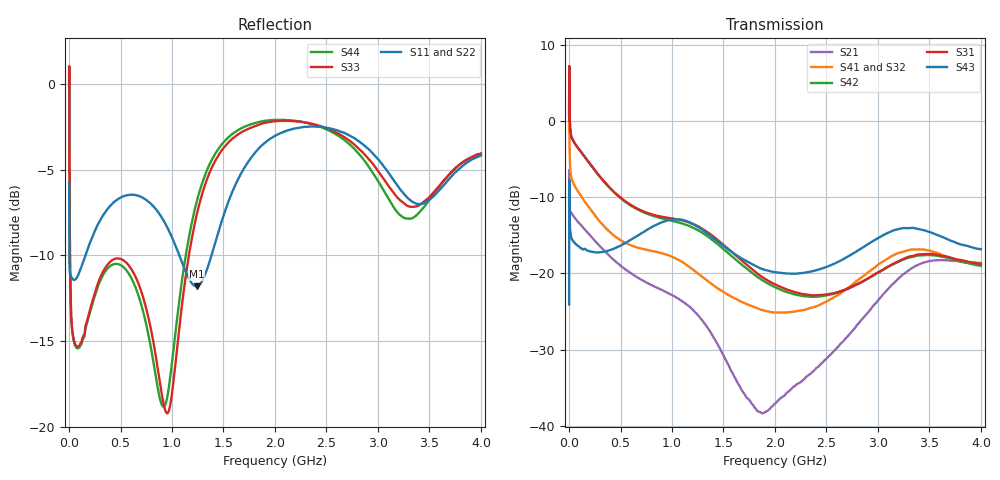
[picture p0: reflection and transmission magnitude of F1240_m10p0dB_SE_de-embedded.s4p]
! Integrated Device Technology
! Corporate Headquarters
! 6024 Silver Creek Valley Road
! San Jose, CA 95138  USA
! Phone:  1-408-284-8200
! Toll Free:  1-800-223-1366
! Webpage:  http://www.idt.com/
! Timing and RF Division
! 515 Groton Road, Suite 102
! Westford, MA 01886-6024
! Device:  F1240
! Description: Dual Intermediate Frequency Digital Variable Gain Amplifier
! Frequency:  10.0 -  500.00 MHz
! Package:  5x5 mm QFN Plastic Package: 32 pin
! Ports:  8 RF, 20 DC
!  Pin  1  = GA3 / Data  Pin 17  = RF OUT_B+
!  Pin  2  = GA4 / CLK  Pin 18  = RF OUT_B-
!  Pin  3  = GA5  Pin 19  = STBY_B
!  Pin  4  = VMODE  Pin 20  = Ground
!  Pin  5  = No Connect  Pin 21  = Ground
!  Pin  6  = GB5  Pin 22  = STB_A
!  Pin  7  = GB4  Pin 23  = RF OUT_A-  = Port 4
!  Pin  8  = GB3  Pin 24  = RF OUT_A+  = Port 3
!  Pin  9  = GB2  Pin 25  = GA0
!  Pin 10  = GB1  Pin 26  = ISET_A
!  Pin 11  = RF IN_B+  Pin 27  = VCC
!  Pin 12  = RF IN_B-  Pin 28  = Ground
!  Pin 13  = Ground  Pin 29  = RF IN_A-  = Port 2
!  Pin 14  = VCC  Pin 30  = RF IN_A+  = Port 1
!  Pin 15  = ISET_B  Pin 31  = GA1
!  Pin 16  = GB0  Pin 32  = GA2 / CSb
! Gain  = +19.5 dB
! State  = 1
! Voltage  = +5.00 V
! Current  = 85.292 mA (one channel only)
! Temperture  =  +25 C
! Test Date  =  2017-10-18
! Board  =  EB4031
! Data:  The device was measured on a custom evaluation board which has
!  individual transmission lines to the RF pins.  Data was collected
!  using a calibrated network analyzer.  The evaluation board was
!  de-embedded using Automatic Fixture Removal.
!  The reference plane is the edge of the package pin.
!  Only Channel A was measured.
!  This data is in single-ended operation.  If your needs are balanced
!  or differential S-parameters then this file needs to be used a
!  linear simulator.
! File Date:  2017-11-10  MJV
! Note:
!  Integrated Device Technology supplies this data as a sample of measured
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# Hz S dB R 100
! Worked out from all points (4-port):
!   410 points, 500 kHz to 4 GHz, reference 100 ohm
!   strongest paths, dB at 500 kHz, 930 MHz, 1.96 GHz, 2.98 GHz, 4 GHz:
!     S43: -24.1, -13.2, -19.7, -15.5, -16.8
!     S31: 0.8, -12.6, -21.2, -20.0, -18.7
!     S42: 0.8, -12.9, -21.5, -20.1, -19.0
!     S41: -1.3, -17.5, -25.1, -19.1, -18.9
!     S32: -1.3, -17.7, -24.9, -19.3, -19.1
!     S21: -6.5, -22.4, -37.6, -23.9, -18.6
!   lowest |S11| = -11.8 dB at 1.24 GHz (marker M1), VSWR 1.69, Z = 60 - j9.88 ohm
!   |S11| at or under -10 dB: 2.973 MHz to 159.4 MHz (156.4 MHz wide, 193 % of centre); 1.071 GHz to 1.383 GHz (311.8 MHz wide, 25.4 % of centre)
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500000  -5.78 -5.6  -6.45 -5.8  -31.83 76.9  -34.09 76.0
        -6.46 -5.8  -5.78 -5.6  -34.04 75.0  -31.83 78.0
        0.84 -111.7  -1.27 -113.4  -0.08 -0.2  -24.09 -37.9
        -1.30 -112.3  0.84 -110.6  -24.09 -37.8  -0.09 2.1
3500000  -10.33 -18.7  -11.23 -17.2  -25.25 3.7  -29.64 -11.4
         -11.23 -17.3  -10.33 -18.8  -29.61 -11.7  -25.25 3.9
         3.14 155.1  -0.91 141.2  -4.17 -82.4  -9.84 177.2
         -0.94 141.5  3.15 155.3  -9.84 177.2  -4.21 -82.4
3.7e8  -7.32 -125.0  -17.42 -99.3  -30.10 -80.4  -37.09 -77.3
       -17.42 -99.3  -7.24 -125.8  -37.19 -75.6  -30.29 -80.5
       -8.38 58.2  -14.32 24.7  -10.57 -161.6  -17.11 50.1
       -14.25 23.9  -8.44 56.9  -17.07 49.9  -10.78 -162.3
1.24e9  -11.80 -162.6  -25.44 102.7  -29.81 120.6  -35.23 152.6
        -25.31 102.5  -11.66 -162.0  -35.01 156.4  -31.14 123.4
        -13.74 -134.6  -19.86 150.3  -7.63 -115.6  -13.96 175.1
        -19.90 143.3  -14.25 -136.0  -13.80 175.4  -6.86 -118.2
2.84e9  -3.46 111.9  -26.13 -10.4  -29.76 -135.7  -32.12 -122.2
        -26.11 -10.6  -3.28 112.4  -32.60 -109.7  -31.06 -127.1
        -21.15 -51.8  -20.78 -128.3  -3.91 104.9  -17.39 -80.0
        -20.55 -139.3  -21.17 -48.2  -16.71 -77.7  -4.25 98.2
3.38e9  -6.99 -3.3  -18.92 -114.1  -26.32 106.2  -28.51 121.7
        -18.94 -114.0  -6.71 0.3  -28.78 136.1  -27.84 114.9
        -17.54 -165.9  -16.89 101.7  -7.13 -19.8  -15.33 167.4
        -16.86 87.5  -17.69 -162.0  -14.14 167.6  -7.63 -36.0
4e9  -4.17 -127.5  -18.64 123.6  -27.29 -19.9  -28.35 -5.0
     -18.64 123.6  -3.94 -126.1  -28.93 8.2  -29.03 -9.3
     -18.74 59.3  -19.13 -35.3  -4.06 -133.0  -18.28 61.4
     -18.86 -49.2  -19.02 65.4  -16.84 55.4  -4.07 -143.0
